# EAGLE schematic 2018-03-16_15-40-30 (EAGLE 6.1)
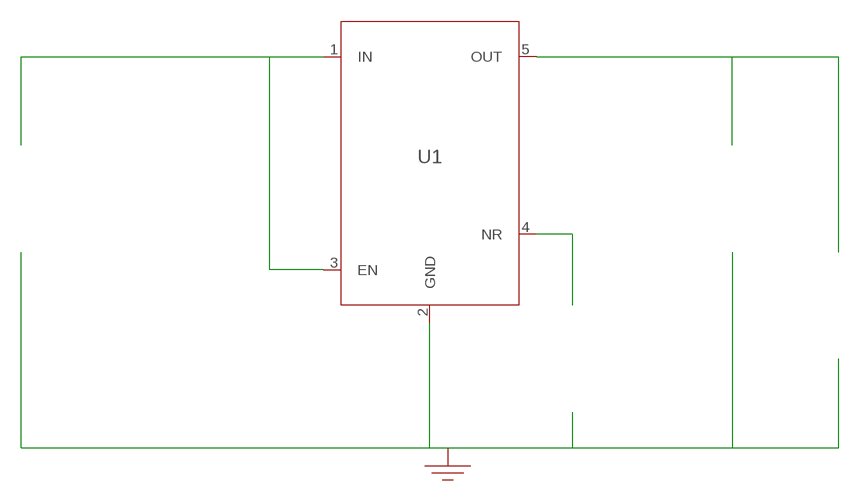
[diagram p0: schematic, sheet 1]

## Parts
CNR  10nF  GRM033R70J103KA01DGRM033R70J103KA01D  [0201]  (not placed on a sheet)
COUT  2.2uF  JMK105BJ225MV-FJMK105BJ225MV-F  [0402]  (not placed on a sheet)
GND  WB_GND  WB_GNDWB_GND  [WB_GND]
IOUT  WB_CURRENT_LOAD  WB_CURRENT_LOADWB_CURRENT_LOAD  [WB_CURRENT_LOAD]  (not placed on a sheet)
U1  TPS79933DDCR  TPS79933DDCRTPS79933DDCR  [R-PDSO-G5]
VIN  WB_BATTERY  WB_BATTERYWB_BATTERY  [WB_BATTERY]  (not placed on a sheet)

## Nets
0: Cnr.1@1 Cout.2@2 GND.1 Iout.-@2 U1.2(GND) Vin.-@2
1: U1.1(IN) U1.3(EN) Vin.+@1
2: Cnr.2@2 U1.4(NR)
3: Cout.1@1 Iout.+@1 U1.5(OUT)
Unconnected: CNR.1 CNR.2 COUT.1 COUT.2 IOUT.1(+) IOUT.2(-) VIN.1(+) VIN.2(-)

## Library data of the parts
CNR = AcceleratedDesigns_Lib:GRM033R70J103KA01D; Cap: 1.0E-8; ESR: 0.0; IRMS: 0.0; Manufacturer_Name: MuRata; Manufacturer_Part_Number: GRM033R70J103KA01D; VDC: 6.3; Vendor: MuRata
COUT = AcceleratedDesigns_Lib:JMK105BJ225MV-F; Cap: 2.2E-6; Datasheet_URL: http://www.yuden.co.jp/productdata/catalog/en/mlcc01%5Fe.pdf; ESR: 0.00152; IRMS: 0.0; Manufacturer_Name: Taiyo Yuden; Manufacturer_Part_Number: JMK105BJ225MV-F; VDC: 6.3; Vendor: Taiyo Yuden
GND = AcceleratedDesigns_Lib:WB_GND; Manufacturer_Name: WB_GND; Manufacturer_Part_Number: WB_GND; PowerPortType: POWER_GROUND; Value: Value
IOUT = AcceleratedDesigns_Lib:WB_CURRENT_LOAD; Manufacturer_Name: WB_CURRENT_LOAD; Manufacturer_Part_Number: WB_CURRENT_LOAD; PowerPortType: POWER_GROUND; Value: Value
U1 = AcceleratedDesigns_Lib:TPS79933DDCR; Datasheet_URL: http://www.ti.com/product/tps79913; Frequency: 0.0; Imax: 0.2; Manufacturer_Name: Texas Instruments; Manufacturer_Part_Number: TPS79913DDCR; Mktg_Package: NA; NSID: TPS79913DDCR; Vendor: Texas Instruments
VIN = AcceleratedDesigns_Lib:WB_BATTERY; Manufacturer_Name: WB_BATTERY; Manufacturer_Part_Number: WB_BATTERY; PowerPortType: POWER_GROUND; Value: Value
